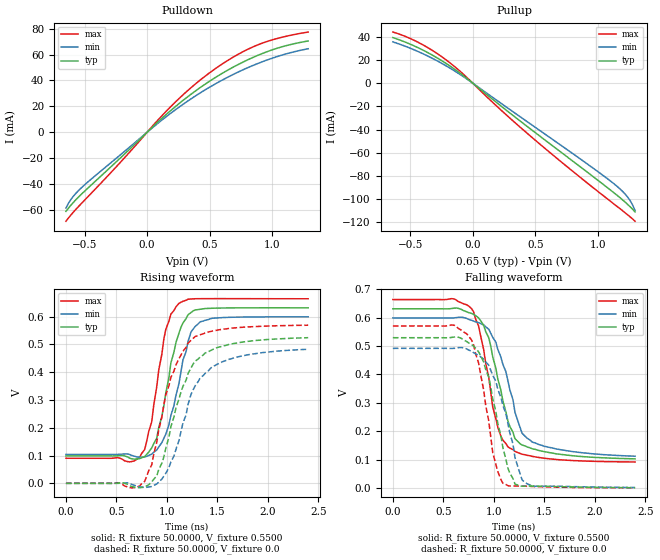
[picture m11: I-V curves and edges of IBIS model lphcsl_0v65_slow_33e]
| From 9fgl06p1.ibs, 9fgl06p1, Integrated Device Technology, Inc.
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[Model]   lphcsl_0v65_slow_33e
Model_type Output
Polarity   Inverting
Enable   Active-High
Vmeas =  0.4000V
Cref =   2.0000pF
Rref =   0.0
Vref =   0.4000V
C_comp   1.1000pF   1.0000pF   1.2000pF
[Temperature Range]   25.0000   85.0000   -40.0000
[Voltage Range]   0.6500V   0.6200V   0.6800V
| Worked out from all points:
|   slope of the pulldown table from 0 to 0.098 V, typ, clamps not added: 10.9 ohm
|   slope of the pullup table from 0 to 0.098 V, typ, clamps not added: 11.3 ohm
|   rising waveform, R_fixture 50.0000, V_fixture 0.5500: 20-80 % time 183ps typ, 191ps min, 151ps max; typ from 0.099 V to 0.632 V
|   rising waveform, R_fixture 50.0000, V_fixture 0.0: 20-80 % time 269ps typ, 285ps min, 254ps max; typ from 0 V to 0.524 V
|   falling waveform, R_fixture 50.0000, V_fixture 0.5500: 20-80 % time 219ps typ, 235ps min, 186ps max; typ from 0.632 V to 0.102 V
|   falling waveform, R_fixture 50.0000, V_fixture 0.0: 20-80 % time 201ps typ, 223ps min, 162ps max; typ from 0.53 V to 0.001 V
[Pulldown]
|Voltage   I(typ)   I(min)   I(max)
-650mV    -61.08mA   -58.52mA   -68.73mA
-630mV    -58.61mA   -54.84mA   -66.21mA
-590mV    -54.11mA   -49.34mA   -61.63mA
-470mV    -42.74mA   -38.03mA   -49.37mA
-210mV    -19.46mA   -17.11mA   -22.79mA
150mV     13.49mA    11.79mA    15.92mA
310mV     26.28mA    23.07mA    30.86mA
450mV     36.16mA    31.86mA    42.2mA
670mV     49.26mA    43.71mA    56.88mA
870mV     58.7mA     52.45mA    66.83mA
1.07V     65.7mA     59.29mA    73.11mA
1.29V     70.48mA    64.48mA    77.38mA
[Pullup]
|Voltage   I(typ)   I(min)   I(max)
-640mV    39.29mA    35.61mA    44.09mA
-500mV    33.59mA    30.11mA    38.48mA
-340mV    25.16mA    22.3mA     29.34mA
-180mV    14.59mA    12.79mA    17.28mA
-40mV     3.496mA    3.04mA     4.187mA
200mV     -17.47mA   -15.35mA   -20.61mA
460mV     -39.31mA   -35.02mA   -45.46mA
1.12V     -93.63mA   -85.83mA   -103.3mA
1.2V      -100.7mA   -93.35mA   -110mA
1.24V     -104.5mA   -98.2mA    -113.5mA
1.28V     -108.7mA   -105mA     -117.1mA
1.3V      -111mA     -109.9mA   -119.1mA
[Ramp]
| variable   typ   min   max
dV/dt_r  0.3146/0.2873n   0.2896/0.3080n   0.3415/0.2476n
dV/dt_f  0.3169/0.2347n   0.2917/0.2676n   0.3433/0.1901n
R_load = 50.0000
[Rising Waveform]
R_fixture= 50.0000
V_fixture= 0.5500
V_fixture_min= 0.5200
V_fixture_max= 0.5800
|time   V(typ)   V(min)   V(max)
0s        98.56mV    104.2mV    90.22mV
730ps     88.87mV    94.2mV     93.79mV
780ps     96.14mV    94.91mV    121.7mV
850ps     127.7mV    105mV      221.5mV
900ps     162.7mV    120.3mV    348.6mV
990ps     327mV      177.4mV    554.8mV
1.12ns    540.8mV    359.7mV    648.1mV
1.24ns    615.1mV    545.3mV    663.5mV
1.33ns    626.6mV    581.5mV    664.6mV
2.4ns     631.7mV    599.4mV    664.3mV
[Rising Waveform]
R_fixture= 50.0000
V_fixture= 0.0
V_fixture_min= 0.0
V_fixture_max= 0.0
|time   V(typ)   V(min)   V(max)
0s        0V         0V         0V
650ps     -11.48mV   -3.424mV   -16.22mV
780ps     -13.53mV   -14.59mV   7.125mV
850ps     4.84mV     -11.14mV   66.49mV
900ps     27.1mV     -2.369mV   148.6mV
1.02ns    165.8mV    56.43mV    350.7mV
1.14ns    329.2mV    186.4mV    462mV
1.28ns    439.8mV    351.1mV    528.3mV
1.62ns    500.7mV    446.9mV    557.7mV
2.4ns     524.3mV    482.6mV    569.2mV
[Falling Waveform]
R_fixture= 50.0000
V_fixture= 0.5500
V_fixture_min= 0.5200
V_fixture_max= 0.5800
|time   V(typ)   V(min)   V(max)
0s        631.7mV    599.5mV    664.2mV
780ps     615.5mV    591.3mV    632.1mV
850ps     599.4mV    582.9mV    570.4mV
950ps     530mV      559.7mV    390.2mV
990ps     461.4mV    530.8mV    284.5mV
1.04ns    384mV      488.3mV    214mV
1.16ns    216.2mV    344.6mV    140.2mV
1.28ns    151.4mV    193mV      118.9mV
1.38ns    138.1mV    161.8mV    111.3mV
2.4ns     102.5mV    111.7mV    91.49mV
[Falling Waveform]
R_fixture= 50.0000
V_fixture= 0.0
V_fixture_min= 0.0
V_fixture_max= 0.0
|time   V(typ)   V(min)   V(max)
0s        529.7mV    492.1mV    571.1mV
610ps     532.2mV    492.3mV    573.4mV
780ps     506.2mV    482mV      521.3mV
850ps     479.8mV    467.9mV    440.4mV
950ps     391.1mV    432.8mV    236.3mV
990ps     313.3mV    396.6mV    123.5mV
1.09ns    142.8mV    291.1mV    16.54mV
1.21ns    13.61mV    107.1mV    6.888mV
1.31ns    6.206mV    18.98mV    6.118mV
2.4ns     876.9uV    1.48mV     371.1uV
